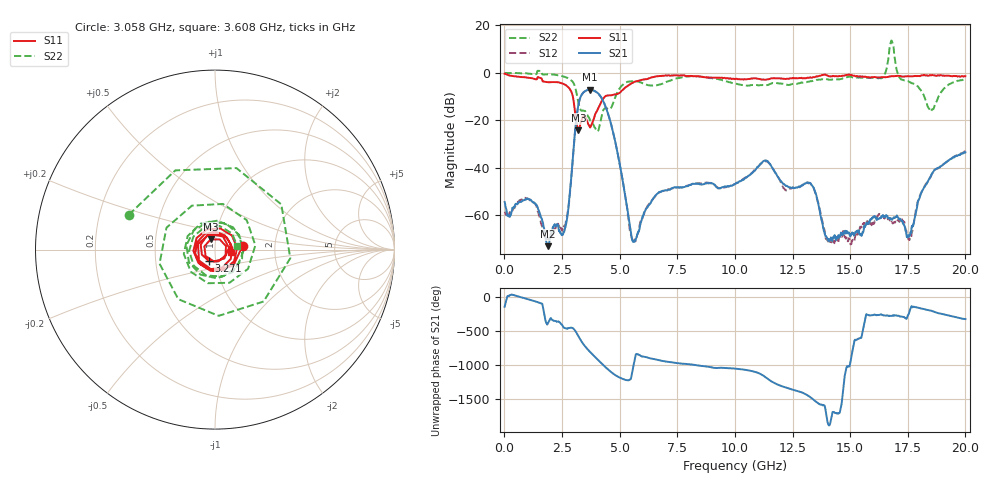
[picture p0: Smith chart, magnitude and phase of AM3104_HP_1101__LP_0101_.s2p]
!Created with skrf (http://scikit-rf.org).
# Hz S RI R 50.0
!freq ReS11 ImS11 ReS21 ImS21 ReS12 ImS12 ReS22 ImS22
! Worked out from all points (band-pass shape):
!   1601 points, 10 MHz to 20 GHz, reference 50 ohm
!   highest |S21| = -7.11 dB at 3.708 GHz (marker M1); lowest = -73.0 dB at 1.884 GHz (marker M2)
!   |S21| within 3 dB of the highest: 3.307 GHz to 4.187 GHz (880.4 MHz wide, 23.5 % of centre)
!   lowest |S11| = -24.2 dB at 3.208 GHz (marker M3), VSWR 1.13, Z = 47.3 + j5.39 ohm
!   |S11| at or under -10 dB: 2.972 GHz to 4.363 GHz (1.391 GHz wide, 37.9 % of centre)
!   |S22| runs from -24.7 to 13.6 dB; largest |S21 - S12| = 0.023
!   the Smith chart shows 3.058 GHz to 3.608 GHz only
!   S11 on the Smith chart (normalised r, x): 3.058 GHz: 1.36, +0.06; 3.271 GHz: 0.93, -0.12; 3.608 GHz: 1.19, -0.04
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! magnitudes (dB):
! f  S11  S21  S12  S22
! 10 MHz  -0.4  -54.4  -58.5  -0.1
! 1.059 GHz  -2.1  -53.2  -53.2  -0.4
! 1.884 GHz  -4.0  -73.0  -69.8  -0.7
! 2.634 GHz  -5.0  -65.1  -64.0  -1.8
! 3.058 GHz  -16.1  -25.4  -25.4  -5.7
! 3.208 GHz  -24.2  -13.7  -13.7  -12.3
! 3.271 GHz  -22.8  -11.1  -11.2  -14.8
! 3.346 GHz  -20.2  -9.3  -9.4  -16.0
! 3.608 GHz  -21.1  -7.3  -7.4  -18.0
! 3.708 GHz  -22.9  -7.1  -7.2  -19.7
! 4.558 GHz  -9.5  -19.1  -19.2  -15.4
! 5.595 GHz  -4.1  -71.1  -70.6  -3.6
! 6.682 GHz  -1.4  -50.5  -50.6  -5.1
! 10.01 GHz  -2.7  -46.9  -46.8  -4.6
! 11.33 GHz  -2.9  -37.0  -37.3  -5.2
! 13.34 GHz  -2.1  -47.3  -47.3  -3.5
! 14.1 GHz  -1.5  -70.6  -72.0  -2.9
! 16.36 GHz  -1.9  -60.4  -59.8  -2.3
! 16.68 GHz  -1.6  -61.3  -61.2  7.1
! 17.6 GHz  -1.5  -68.0  -69.3  -4.0
! 18.49 GHz  -1.0  -43.7  -44.0  -16.3
! 20 GHz  -1.4  -33.5  -33.0  -2.7
